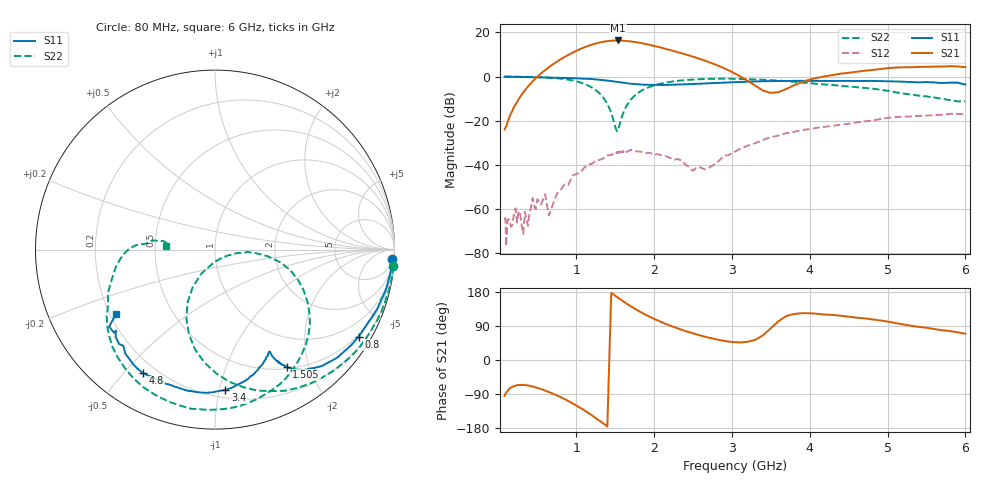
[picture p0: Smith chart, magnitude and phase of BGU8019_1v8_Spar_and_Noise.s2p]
! BGU8019,  Vcc= 1.80 V, Icc= 4.3800 mA
# MHz S MA R 50
!  Freq-MHz  S11-mag  S11-arg  S21-mag  S21-arg  S12-mag  S12-arg  S22-mag  S22-arg
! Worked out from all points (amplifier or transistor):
!   130 points, 80 MHz to 6 GHz, reference 50 ohm
!   highest |S21| = 16.3 dB at 1.54 GHz (marker M1)
!   |S21| within 3 dB of that: 1.112 GHz to 2.066 GHz (953.6 MHz wide, 60 % of centre)
!   unconditionally stable (mu >= 1): start of sweep to 124.4 MHz; 150.8 MHz to 277.9 MHz; 283.5 MHz to end of sweep
!   at 480 MHz: K = 2.58, MAG = 22.7 dB, |S12| = -60.0 dB
!   at 1.615 GHz: K = 1.80, MAG = 20.0 dB, |S12| = -34.2 dB
!   at 6 GHz: K = 1.42, MAG = 6.9 dB, |S12| = -17.2 dB
!   lowest NFmin = 0.40 dB at 1 GHz
!   S11 on the Smith chart (normalised r, x): 80 MHz: 7, -35; 800 MHz: 0.45, -3.52; 1.505 GHz: 0.53, -1.66; 3.4 GHz: 0.26, -1.04; 4.8 GHz: 0.15, -0.57; 6 GHz: 0.22, -0.28
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80  0.9886 -3.2  0.06339 -94.7  0.0005839 19.5  0.9975 -5.3
100  0.9898 -4.1  0.07446 -86.7  0.0001463 111.0  0.9968 -6.5
120  0.9888 -5.0  0.09551 -81.3  0.0005865 -29.8  0.997 -8.1
220  0.9827 -9.1  0.2324 -67.7  0.001049 158.1  0.9928 -14.8
320  0.978 -13.1  0.439 -65.7  0.0002777 95.4  0.9875 -21.5
440  0.9669 -17.8  0.7796 -70.0  0.001789 -115.2  0.9762 -30.2
600  0.9497 -23.8  1.399 -80.6  0.002188 173.6  0.9527 -42.2
650  0.9452 -25.6  1.639 -84.6  0.0007181 151.6  0.942 -46.2
800  0.9359 -31.2  2.458 -98.0  0.002739 -129.7  0.8979 -59.0
1100  0.9003 -43.2  4.552 -132.2  0.00858 -176.6  0.6883 -89.5
1300  0.8456 -51.9  5.879 -160.4  0.01304 158.2  0.4174 -112.5
1505  0.766 -58.5  6.521 169.0  0.01979 132.2  0.07015 -94.0
1540  0.7512 -59.3  6.548 163.8  0.01913 125.2  0.06394 -41.7
1800  0.6647 -61.7  5.859 129.6  0.02014 92.1  0.4336 -15.2
2100  0.6443 -62.2  4.47 99.5  0.01637 58.2  0.7021 -42.0
2500  0.6777 -66.0  2.815 70.3  0.007366 -15.5  0.8544 -71.2
3100  0.7545 -78.2  1.027 46.4  0.02289 -134.5  0.8858 -106.8
3400  0.784 -85.8  0.4815 65.1  0.037 -159.4  0.8488 -122.4
4100  0.7975 -104.1  0.942 121.8  0.06986 163.1  0.6798 -151.5
4800  0.7969 -120.2  1.403 107.3  0.1015 141.6  0.5342 -173.8
5100  0.7748 -127.8  1.596 97.7  0.1212 129.2  0.4414 176.8
6000  0.6594 -146.9  1.63 69.1  0.1384 102.8  0.2745 175.4
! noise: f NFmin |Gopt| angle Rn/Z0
1000  0.3974  0.6454  31.59  0.196
1250  0.4459  0.6104  34.05  0.1888
1505  0.5214  0.5739  43.36  0.188
1535  0.5117  0.5853  43.96  0.1923
1560  0.5192  0.5873  43.78  0.1897
1590  0.5069  0.5772  43.89  0.1889
1620  0.4988  0.5766  46.04  0.1923
1645  0.5413  0.5768  45.81  0.1869
1900  0.5999  0.5644  51.44  0.201
2200  0.6417  0.5115  60.17  0.1924
